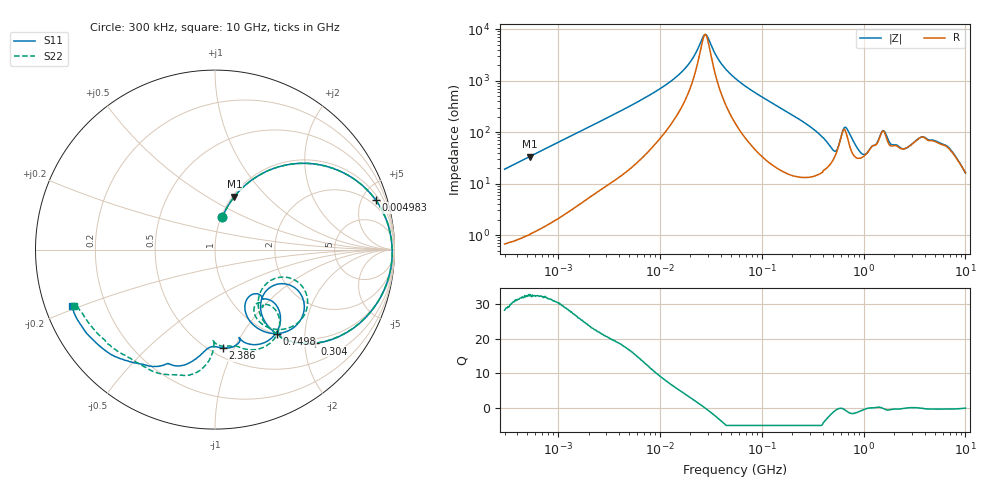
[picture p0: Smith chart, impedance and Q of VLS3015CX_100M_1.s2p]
! S-Parameter Data Generated by TDK Corporation
! Copyright(C) 2019 TDK Corporation.
! All Rights Reserved.
! TDK P/N: VLS3015CX-100M-1 (Inductor)
! Property: L=10uH at 1MHz
! Size(LxWxT): 3x3x1.5mm
! Model Type: s2p (Touchstone File Format Version 1.0)
! Frequency: DC=Yes Start=0.3MHz Stop=10000MHz 802points Log-sweep
! Model Generated on Sep. 23, 2019
! Port Assignments:
!  1 ---@@@--- 2
! Applicable Conditions:
!  Temperature = 25 degC
!  DC Bias Current = 0 A
!  Small Signal Operation
! Terms and conditions regarding TDK Simulation Models
! (1)This simulation model is being provided solely for informational purposes. Please refer to the specifications of the products in terms of detailed characteristics of such products.
! (2)In no event shall TDK Corporation of any of its subsidiaries be liable for any loss or damage arising, directly or indirectly,
!  From any information contained in this simulation model, including, but not limited to loss or damages arising from any inaccuracies, omissions or errors in connection with such information.
! (3)Any and all copyrights on this simulation model are owned by TDK Corporation.
!  Duplication or redistribution of this simulation model without prior written permission from TDK Corporation is prohibited.
! (4)This simulation model is subject to any modification or change without any prior notice.
! (5)Neither TDK Corporation nor any of its subsidiaries shall make any warranty, express or implied,
!  Including but not limited to the correctness, implied warranties of merchantability and fitness for a particular purpose with respect to this simulation models.
! (6)The use of this simulation model shall be deemed to have consented to the terms and conditions hereof.
# Hz S MA R 50
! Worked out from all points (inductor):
!   801 points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, 300 kHz to 10 GHz, reference 50 ohm
!   read as one part in series: L = 10.1 uH near 318.3 kHz
!   highest Q = 32.4 at 529.7 kHz (marker M1), where L = 10.1 uH
!   self-resonance near 27.95 MHz
!   S11 on the Smith chart (normalised r, x): 300 kHz: 1.01, +0.38; 4.983 MHz: 1.39, +6.29; 304 MHz: 0.89, -2.22; 749.8 MHz: 1.02, -1.44; 2.386 GHz: 0.57, -0.90; 10 GHz: 0.08, -0.19
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300000  0.1854 77.2  0.976 -10.7  0.9762 -10.7  0.1851 77.3
529652  0.3144 69.9  0.9398 -18.4  0.9397 -18.4  0.3142 69.9
1713600  0.7167 42.0  0.6697 -45.8  0.6698 -45.8  0.7166 42.0
4982740  0.9365 17.3  0.2995 -69.3  0.2995 -69.3  0.9365 17.3
9671944  0.9739 8.2  0.1472 -75.9  0.1473 -75.9  0.974 8.2
1.80882e7  0.9849 2.5  0.05458 -73.0  0.0546 -73.0  0.985 2.5
2.78833e7  0.9874 -0.8  0.01254 -2.0  0.01255 -2.0  0.9874 -0.7
5.477226e7  0.9842 -6.5  0.0881 75.7  0.08813 75.7  0.9842 -6.5
1.540638e8  0.9307 -22.5  0.3137 64.1  0.3137 64.1  0.9306 -22.3
3.040112e8  0.7622 -43.3  0.5748 40.9  0.5748 40.9  0.7614 -43.2
3.126428e8  0.7498 -44.3  0.5869 39.6  0.5869 39.6  0.7489 -44.2
4.866838e8  0.4373 -53.8  0.7294 9.7  0.7294 9.7  0.4253 -54.5
5.82867e8  0.4167 -27.1  0.6029 -9.3  0.6029 -9.3  0.3898 -23.4
6.573376e8  0.6015 -34.4  0.4426 1.7  0.4427 1.6  0.5926 -29.4
7.497801e8  0.581 -53.6  0.5779 11.1  0.5779 11.1  0.5899 -48.5
1.165098e9  0.3392 -46.5  0.6465 -22.4  0.6464 -22.4  0.3975 -48.9
1.525386e9  0.5392 -47.4  0.4511 -32.4  0.4509 -32.4  0.5583 -49.9
1.767019e9  0.5528 -71.1  0.5208 -21.9  0.5205 -21.8  0.5823 -72.6
2.38587e9  0.5496 -85.5  0.5488 -39.1  0.5487 -39.1  0.5144 -90.6
4.865898e9  0.7073 -114.2  0.3171 -67.1  0.3176 -67.2  0.7537 -113.1
7.06055e9  0.8078 -131.5  0.258 -82.1  0.2576 -82.2  0.7907 -137.6
1e10  0.8571 -158.7  0.2108 -94.1  0.2106 -94.0  0.8453 -158.3
